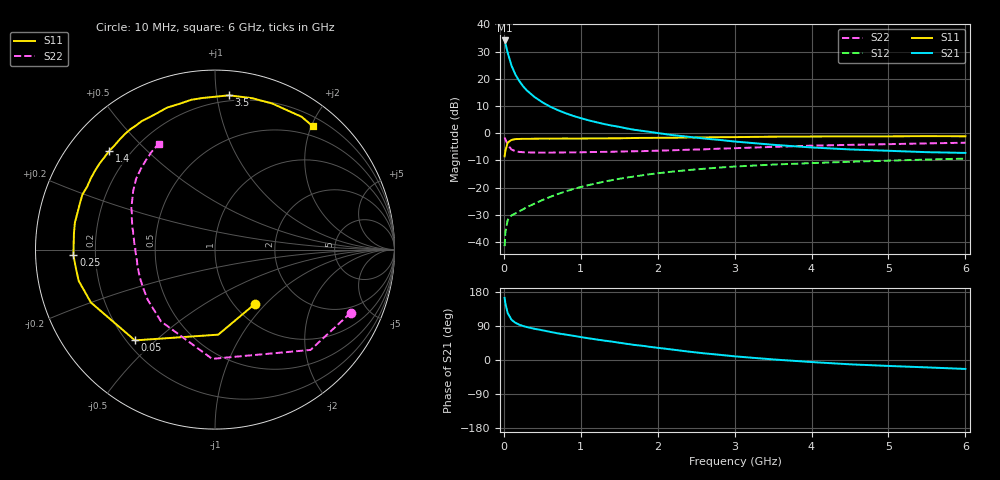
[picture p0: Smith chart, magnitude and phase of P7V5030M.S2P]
! SIEMENS Small Signal Semiconductors
! BFP196
! Si NPN RF Bipolar Junction Transistor in SOT143
! VCE = 0.5 V  IC = 30 mA
! Common Emitter S-Parameters:  May  1996
# GHz  S  MA  R  50
!  f  S11  S21  S12  S22
! GHz  MAG  ANG  MAG  ANG  MAG  ANG  MAG  ANG
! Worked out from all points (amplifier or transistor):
!   36 points, 10 MHz to 6 GHz, reference 50 ohm
!   highest |S21| = 34.1 dB at 10 MHz (marker M1)
!   |S21| within 3 dB of that: start of sweep to 36.89 MHz
!   unconditionally stable (mu >= 1): 452.5 MHz to end of sweep
!   at 250 MHz: K = 0.78, MSG = 22.6 dB, |S12| = -28.0 dB
!   at 1.4 GHz: K = 1.15, MAG = 7.7 dB, |S12| = -17.3 dB
!   at 6 GHz: K = 1.05, MAG = -0.4 dB, |S12| = -9.3 dB
!   S11 on the Smith chart (normalised r, x): 10 MHz: 1.23, -0.87; 50 MHz: 0.23, -0.43; 250 MHz: 0.12, -0.02; 1.4 GHz: 0.12, +0.39; 3.5 GHz: 0.16, +1.08; 6 GHz: 0.34, +2.03
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0.01  0.3755 -53.7  50.56 163.9  0.0084 74.7  0.8338 -25.0
0.02  0.4742 -87.8  44.84 149.2  0.015 62.5  0.7719 -46.4
0.05  0.6743 -131.4  30.05 123.6  0.0255 43.2  0.6089 -91.5
0.1  0.7517 -156.9  17.39 106.2  0.0309 35.4  0.5004 -127.0
0.15  0.7792 -167.1  11.98 98.2  0.0337 36.3  0.4675 -143.3
0.2  0.7825 -173.0  9.123 93.2  0.0366 39.1  0.4531 -152.4
0.25  0.7896 -177.8  7.282 89.7  0.0399 42.3  0.4472 -158.6
0.3  0.788 178.7  6.091 86.9  0.0438 44.8  0.4439 -162.5
0.4  0.7913 173.2  4.612 82.3  0.0509 49.4  0.4415 -168.3
0.5  0.7949 169.1  3.703 78.5  0.059 51.6  0.4392 -172.0
0.6  0.7932 164.9  3.089 74.3  0.0673 53.4  0.4396 -174.7
0.7  0.7959 160.8  2.66 70.4  0.076 54.3  0.4418 -177.0
0.9  0.794 154.0  2.083 64.0  0.0939 54.2  0.4442 179.3
1.1  0.7998 147.0  1.727 57.3  0.1112 53.4  0.4488 176.5
1.4  0.8062 137.1  1.38 48.7  0.1367 50.2  0.456 172.4
1.7  0.8165 127.9  1.154 39.7  0.1607 46.5  0.4654 168.4
2.2  0.824 114.3  0.92 27.3  0.1974 39.1  0.4857 162.0
2.8  0.8452 98.9  0.753 13.8  0.2335 30.3  0.5196 153.7
3.5  0.8628 84.9  0.613 1.5  0.265 20.2  0.5602 144.5
4.5  0.8742 68.6  0.503 -11.4  0.2986 8.3  0.6103 132.7
5.5  0.8835 56.9  0.448 -19.5  0.3279 -2.2  0.6496 122.9
6  0.877 51.5  0.434 -23.6  0.3414 -7.9  0.6681 117.9
